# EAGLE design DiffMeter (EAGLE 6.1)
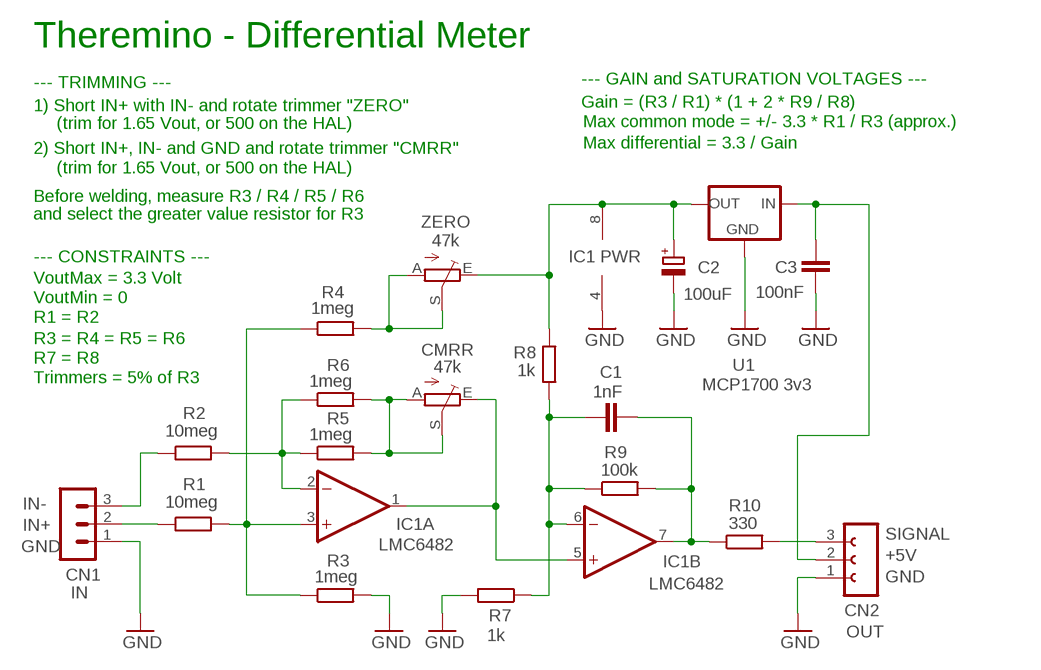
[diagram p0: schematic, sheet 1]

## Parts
C1  1nF  C-EU025-024X044  [C025-024X044]
C2  100uF  CPOL-EUE2-5B  [E2-5B]
C3  100nF  C-EU025-024X044  [C025-024X044]
CMRR  47k  TRIMMERTRIM_M2  [TRIM_M2]
CN1  IN  MA03-1N  [MA03-1]
CN2  OUT  FE03-1"  [FE03-1]
IC1  LMC6482  TL072P  [DIL08]
R1  10meg  R-EU_0204/5  [0204/5]
R2  10meg  R-EU_0204/5  [0204/5]
R3  1meg  R-EU_0204/5  [0204/5]
R4  1meg  R-EU_0204/5  [0204/5]
R5  1meg  R-EU_0204/5  [0204/5]
R6  1meg  R-EU_0204/5  [0204/5]
R7  1k  R-EU_0204/5  [0204/5]
R8  1k  R-EU_0204/5  [0204/5]
R9  100k  R-EU_0204/5  [0204/5]
R10  330  R-EU_0204/5  [0204/5]
U1  MCP1700 3v3  MCP1700L1  [TO92L1]
ZERO  47k  TRIMMERTRIM_M2  [TRIM_M2]

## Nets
GND: C2.- C3.2 CN1.1 CN2.1 IC1.4(P:V-) R3.2 R7.2 U1.3(GND)
N$1: IC1.2(A:-IN) R2.2 R5.1 R6.1
N$2: C1.1 IC1.6(B:-IN) R7.1 R8.2 R9.1
N$3: R4.2 ZERO.A ZERO.S
N$4: IC1.3(A:+IN) R1.2 R3.1 R4.1
N$5: C1.2 IC1.7(B:OUT) R9.2 R10.1
N$6: CMRR.E IC1.1(A:OUT) IC1.5(B:+IN)
N$7: CN2.3 R10.2
N$8: C3.1 CN2.2 U1.2(IN)
N$9: CN1.2 R1.1
N$10: C2.+ IC1.8(P:V+) R8.1 U1.1(OUT) ZERO.E
N$11: CN1.3 R2.1
N$16: CMRR.A CMRR.S R5.2 R6.2

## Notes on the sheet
- Theremino - Differential Meter
- --- TRIMMING --- | --- GAIN and SATURATION VOLTAGES ---
- 1) Short IN+ with IN- and rotate trimmer "ZERO" | Gain = (R3 / R1) * (1 + 2 * R9 / R8)
- (trim for 1.65 Vout, or 500 on the HAL) | Max common mode = +/- 3.3 * R1 / R3 (approx.)
- Max differential = 3.3 / Gain
- 2) Short IN+, IN- and GND and rotate trimmer "CMRR"
- (trim for 1.65 Vout, or 500 on the HAL)
- Before welding, measure R3 / R4 / R5 / R6
- and select the greater value resistor for R3
- --- CONSTRAINTS --- | IC1 PWR
- VoutMax = 3.3 Volt
- VoutMin = 0
- R1 = R2
- R3 = R4 = R5 = R6
- R7 = R8
- Trimmers = 5% of R3
- IN-
- IN+
- SIGNAL
- GND
- +5V
- GND

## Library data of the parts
C1 C3 = 00-LIVIO:C-EU: CAPACITOR, European symbol
C2 = 00-LIVIO:CPOL-EU: POLARIZED CAPACITOR, European symbol
CMRR ZERO = 00-LIVIO:TRIMMER: Horizzontal and Vertical trimmers
CN1 = 03-con-lstb-M:MA03-1: PIN HEADER
CN2 = 02-con-lsta-F:FE03-1: FEMALE HEADER
IC1 = linear:TL072: OP AMP
R1-R10 = 00-LIVIO:R-EU_: RESISTOR, European symbol
U1 = 00-LIVIO:MCP1700: Linear regulator Quescient courrent 1.8uA Input 2.3v to 6v Output 1.2v 1.8v 2.5v 3.0v 3.3v 5.0v

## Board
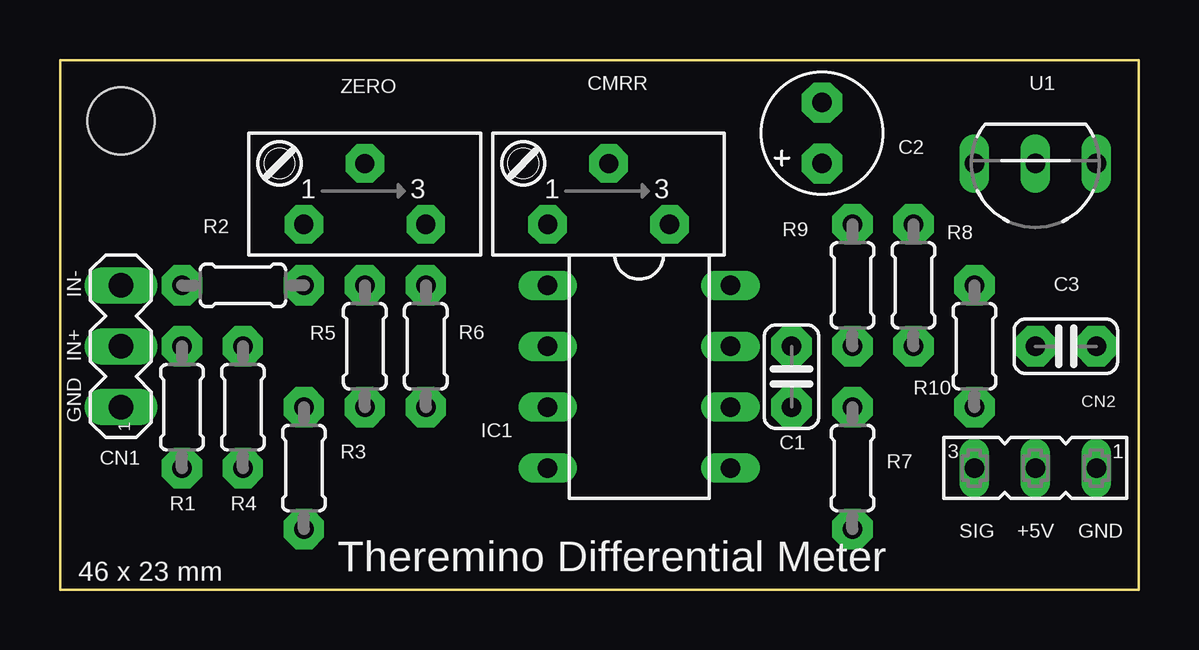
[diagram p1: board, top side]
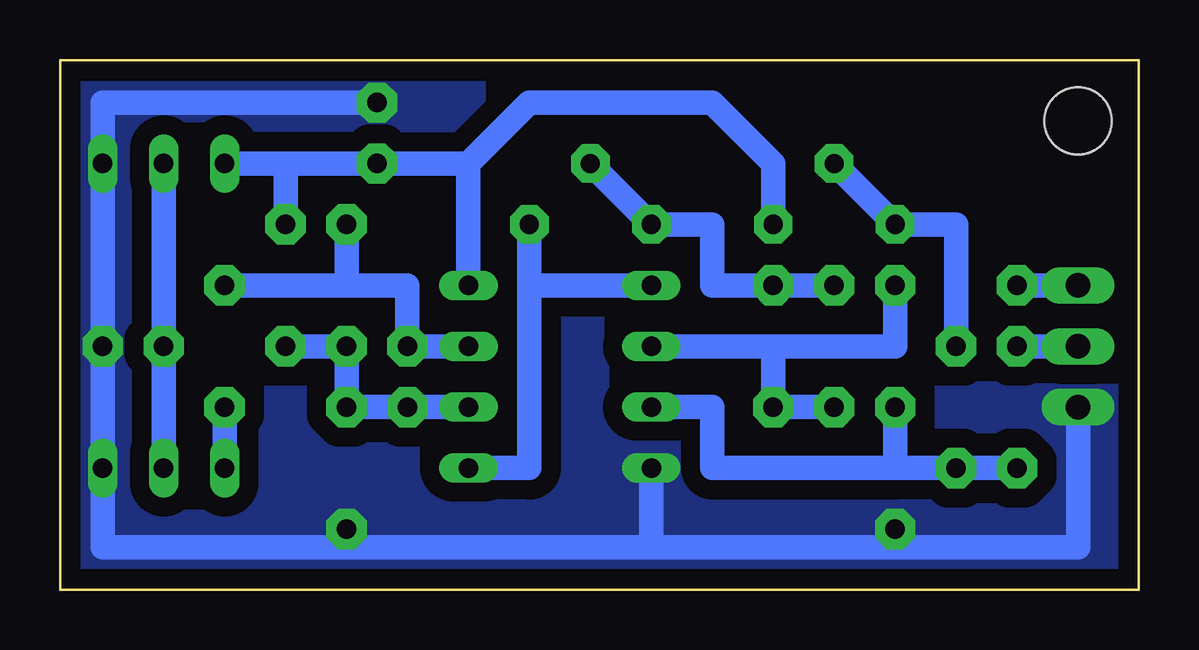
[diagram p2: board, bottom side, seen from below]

Size 44.96 x 22.1 mm. Coordinates in mm from the lower left corner, seen from the top.
Outline: 0,0 44.96,0 44.96,22.1 0,22.1 0,0
Copper layers (1*16): Top 0.035mm / dielectric 1.5mm / Bottom 0.035mm
Design rules: minimum track width 10mil, minimum drill 0.6mm, track to track 8mil, track to pad 8mil, pad to pad 8mil, via to via 8mil, smd to smd 8mil, copper to edge 31mil, drill to drill 8mil, minimum pad ring 5mil, minimum via ring 8mil, stop-mask expansion 4mil, vias tented up to drill 0mil, thermal gap 41mil
Holes 2.8 mm at 2.54,19.56

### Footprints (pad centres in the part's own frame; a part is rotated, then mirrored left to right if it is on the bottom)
C025-024X044 = drill 0.813 pad 1.676 octagon: 1 -1.27,0; 2 1.27,0
E2-5B = drill 0.813 pad 1.676 octagon: + -1.27,0; - 1.27,0
TRIM_M2 = drill 0.8 pad 1.6 octagon: A 2.54,2.54; E -2.54,2.54; S 0,0
MA03-1 = drill 1.016 long: 1 -2.54,0; 2 0,0; 3 2.54,0
FE03-1 = drill 0.813 long: 1 -2.54,0; 2 0,0; 3 2.54,0
DIL08 = drill 0.813 long: 1 -3.81,-3.81; 2 -1.27,-3.81; 3 1.27,-3.81; 4 3.81,-3.81; 5 3.81,3.81; 6 1.27,3.81; 7 -1.27,3.81; 8 -3.81,3.81
0204/5 = drill 0.813 pad 1.676 octagon: 1 -2.54,0; 2 2.54,0
TO92L1 = drill 0.813 long: 1 2.54,0; 2 0,0; 3 -2.54,0

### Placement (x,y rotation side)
C1  30.48,8.89 90 top
C2  31.75,19.05 90 top
C3  41.91,10.16 0 top
CMRR  22.86,17.78 180 top
CN1  2.54,10.16 90 top
CN2  40.64,5.08 180 top
IC1  24.13,8.89 270 top
R1  5.08,7.62 270 top
R2  7.62,12.7 0 top
R3  10.16,5.08 270 top
R4  7.62,7.62 90 top
R5  12.7,10.16 90 top
R6  15.24,10.16 90 top
R7  33.02,5.08 270 top
R8  35.56,12.7 270 top
R9  33.02,12.7 90 top
R10  38.1,10.16 270 top
U1  40.64,17.78 180 top
ZERO  12.7,17.78 180 top

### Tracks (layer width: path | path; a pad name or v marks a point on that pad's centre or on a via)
GND
  Bottom 1.016: 20.32,1.78 IC1.4 | 10.16,1.78 2.54,1.78 CN1.1 | 10.16,1.78 R3.2 10.16,1.78 | 10.16,1.78 20.32,1.78 | 20.32,1.78 33.02,1.78 | 33.02,1.78 R7.2 33.02,1.78 | 33.02,1.78 43.18,1.78 CN2.1 43.18,9.14 C3.2 U1.3 43.18,20.32 C2.-
  pour Bottom (isolate 0.8, rank 6, no thermals): -1,-1 45.96,-1 45.96,23.1 -1,23.1
N$1
  Bottom 1.016: R5.1 R6.1 15.24,10.16 | 15.24,10.16 IC1.2 | 15.24,10.16 10.16,10.16 R2.2
N$2
  Bottom 1.016: IC1.6 C1.1 R7.1 | R9.1 R7.1 | R8.2 R9.1 | R9.1 R7.1
N$3
  Bottom 1.016: ZERO.S ZERO.A 7.62,15.24 7.62,10.41 R4.2
N$4
  Bottom 1.016: IC1.3 17.78,7.62 17.78,5.08 10.16,5.08 | R1.2 R4.1 10.16,5.08 | 10.16,5.08 R3.1 10.16,5.08
N$5
  Bottom 1.016: IC1.7 C1.2 30.48,11.43 30.48,12.7 33.02,12.7 | 33.02,12.7 34.29,12.7 35.56,12.7 R10.1 | R9.2 33.02,12.7
N$6
  Bottom 1.016: IC1.5 25.4,5.08 25.4,12.7 | IC1.1 25.4,12.7 | 25.4,12.7 CMRR.E
N$7
  Bottom 1.016: R10.2 CN2.3
N$8
  Bottom 1.016: U1.2 C3.1 CN2.2
N$9
  Bottom 1.016: CN1.2 R1.1
N$10
  Bottom 1.016: ZERO.E 15.24,17.78 17.78,20.32 25.4,20.32 27.94,17.78 | 35.56,17.78 C2.+ 27.94,17.78 | 35.56,17.78 U1.1 | IC1.8 27.94,17.78 | R8.1 35.56,17.78 | 35.56,17.78 U1.1 | U1.1 35.56,17.78
N$11
  Bottom 1.016: CN1.3 R2.1
N$16
  Bottom 1.016: CMRR.S CMRR.A 17.78,15.24 17.78,12.7 R6.2 R5.2

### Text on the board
tNames: IN- | IN+ | GND | SIG | +5V | GND | Theremino Differential Meter | 46 x 23 mm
